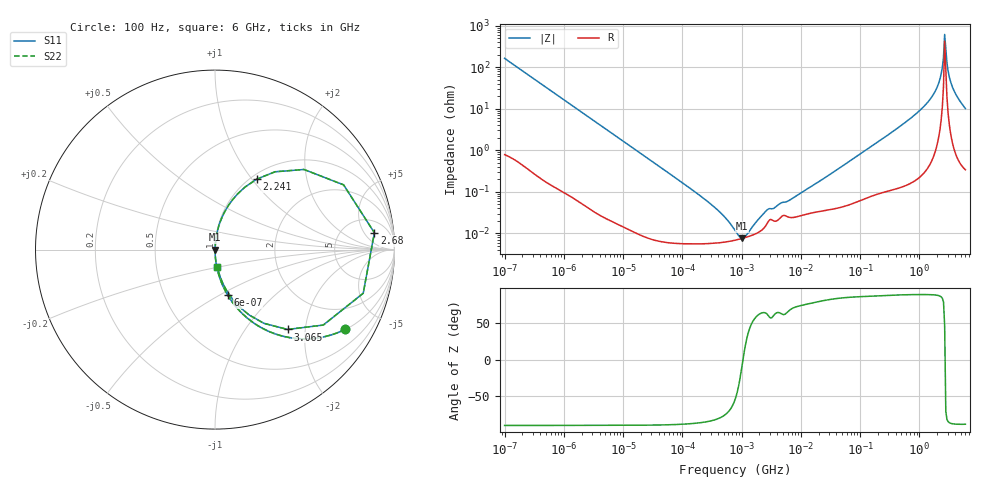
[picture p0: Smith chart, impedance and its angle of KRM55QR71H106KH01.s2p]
!Murata Part Number: KRM55QR71H106KH01
!These Parameters are Measured in Series Mode Connection
!Data Generated on Jan 08, 2026
!  o--ll--o
!Port1  Port2
!  o------o
!Operation Temp=25[degC], DC Bias Voltage=0[V]
!Freq. Start=100[Hz] Stop=6[GHz] 401[Steps]
# Hz S RI R 50
!Freq.(Hz) S11(Real) S11(Imag) S21(Real) S21(Imag) S12(Real) S12(Imag) S22(Real) S22(Imag)
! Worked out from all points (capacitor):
!   401 points, 100 Hz to 6 GHz, reference 50 ohm
!   read as one part in series: C = 9.74 uF near 109 Hz
!   lowest |Z| = 7.62 mohm at 1.013 MHz (marker M1)
!   series resonance near 1.057 MHz, so ESL is about 2.3 nH
!   S11 on the Smith chart (normalised r, x): 100 Hz: 1.02, -3.26; 600 Hz: 1.00, -0.55; 2.241 GHz: 1.07, +1.05; 2.68 GHz: 10, +9; 3.065 GHz: 1.15, -1.61; 6 GHz: 1.01, -0.20
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100  0.7258 -0.4437  0.2742 0.4437  0.2742 0.4437  0.7258 -0.4437
205  0.3903 -0.4851  0.6097 0.4851  0.6097 0.4851  0.3903 -0.4851
600  0.0709 -0.254  0.9291 0.254  0.9291 0.254  0.0709 -0.254
2008  0.0072 -0.0815  0.9928 0.0815  0.9928 0.0815  0.0072 -0.0815
40335  8.15e-05 -0.00412  0.9999 0.00412  0.9999 0.00412  8.15e-05 -0.00412
316350  5.75e-05 -0.000476  0.9999 0.000476  0.9999 0.000476  5.75e-05 -0.000476
774597  6.83e-05 -9.65e-05  0.9999 9.65e-05  0.9999 9.65e-05  6.83e-05 -9.65e-05
1013323  7.51e-05 -1.27e-05  0.9999 1.27e-05  0.9999 1.27e-05  7.51e-05 -1.27e-05
1325623  8.43e-05 6.85e-05  0.9999 -6.85e-05  0.9999 -6.85e-05  8.43e-05 6.85e-05
2713602  0.000174 0.000324  0.9998 -0.000324  0.9998 -0.000324  0.000174 0.000324
1.555665e7  0.000313 0.00135  0.9997 -0.00135  0.9997 -0.00135  0.000313 0.00135
3.124326e8  0.00166 0.0246  0.9983 -0.0246  0.9983 -0.0246  0.00166 0.0246
1.251881e9  0.0174 0.1188  0.9826 -0.1188  0.9826 -0.1188  0.0174 0.1188
1.873145e9  0.0757 0.2473  0.9243 -0.2473  0.9243 -0.2473  0.0757 0.2473
2.240541e9  0.2319 0.3921  0.7681 -0.3921  0.7681 -0.3921  0.2319 0.3921
2.450438e9  0.4957 0.4464  0.5043 -0.4464  0.5043 -0.4464  0.4957 0.4464
2.679998e9  0.8882 0.0936  0.1118 -0.0936  0.1118 -0.0936  0.8882 0.0936
2.931063e9  0.6034 -0.4203  0.3966 0.4203  0.3966 0.4203  0.6034 -0.4203
3.065283e9  0.4043 -0.445  0.5957 0.445  0.5957 0.445  0.4043 -0.445
3.352442e9  0.19 -0.3642  0.81 0.3642  0.81 0.3642  0.19 -0.3642
3.666503e9  0.1031 -0.2828  0.8969 0.2828  0.8969 0.2828  0.1031 -0.2828
6e9  0.0134 -0.0993  0.9866 0.0993  0.9866 0.0993  0.0134 -0.0993
